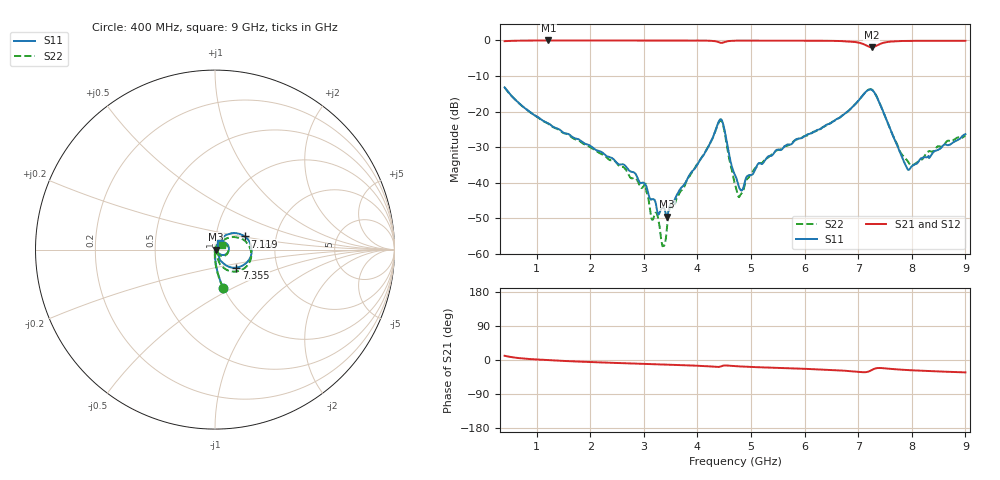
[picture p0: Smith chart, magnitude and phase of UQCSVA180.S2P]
!  Part Number  UQCSVA180  Mounting Orientation: Horizontal
!  Description: Ultra Low ESR Microwave capacitors
!  Application: Coupling, Bypass, Tuning, DC Block
!  Filters, Matching
# GHZ S DB R 50
! Freq  |S11|  S11 Ph  |S21|  S21 Ph  |S12|  S12 Ph  |S22|  S22 Ph
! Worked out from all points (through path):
!   801 points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, 400 MHz to 9 GHz, reference 50 ohm
!   highest |S21| = -0.04 dB at 1.217 GHz (marker M1); lowest = -2.0 dB at 7.248 GHz (marker M2)
!   group delay of S21, straight-line fit = 11.7 ps
!   lowest |S11| = -49.5 dB at 3.432 GHz (marker M3), VSWR 1.01, Z = 50.3 + j0.0271 ohm
!   |S11| at or under -10 dB: start of sweep to end of sweep
!   |S22| runs from -57.8 to -13.2 dB; largest |S21 - S12| = 0.01
!   S11 on the Smith chart (normalised r, x): 400 MHz: 1.00, -0.45; 7.119 GHz: 1.38, +0.21; 7.355 GHz: 1.24, -0.25; 9 GHz: 1.05, +0.08
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0.4  -13.21 -77.5  -0.24 11.2  -0.27 11.2  -13.24 -78.0
1.217  -23.31 -87.4  -0.04 -0.6  -0.08 -0.5  -23.46 -88.2
1.841  -28.44 -89.0  -0.04 -4.5  -0.07 -4.4  -28.75 -91.1
3.012  -40.25 -102.6  -0.04 -10.2  -0.08 -10.1  -40.52 -78.9
3.141  -44.67 -58.1  -0.04 -10.9  -0.07 -10.8  -49.96 -77.9
3.27  -48.93 -34.8  -0.05 -11.4  -0.08 -11.4  -50.38 -41.7
3.356  -47.01 -20.9  -0.05 -11.8  -0.08 -11.8  -57.79 18.0
3.432  -49.50 4.6  -0.05 -12.2  -0.08 -12.2  -52.28 19.3
3.496  -45.90 33.5  -0.04 -12.5  -0.08 -12.5  -46.83 39.8
4.152  -31.22 60.5  -0.09 -16.2  -0.13 -16.1  -31.06 58.8
4.421  -22.23 14.8  -0.66 -17.6  -0.70 -17.5  -22.56 5.7
4.496  -24.55 -30.1  -0.53 -14.6  -0.57 -14.4  -25.02 -41.0
4.7  -37.81 -27.1  -0.10 -16.2  -0.15 -16.0  -40.49 -39.5
4.818  -42.16 16.9  -0.08 -17.1  -0.12 -16.9  -43.03 18.9
5.141  -34.53 60.0  -0.08 -19.1  -0.11 -18.9  -34.73 54.9
6.141  -25.99 64.2  -0.11 -24.1  -0.13 -23.8  -25.87 51.2
7.119  -14.83 23.9  -1.20 -32.3  -1.25 -32.0  -14.84 12.1
7.248  -13.85 -10.2  -1.97 -26.9  -2.02 -26.6  -13.80 -21.7
7.355  -16.19 -40.2  -1.37 -21.3  -1.43 -21.0  -16.11 -51.4
7.57  -23.91 -64.1  -0.42 -23.0  -0.48 -22.6  -23.82 -72.5
7.936  -36.39 -21.3  -0.17 -26.7  -0.21 -26.4  -34.20 -30.8
9  -26.33 54.8  -0.14 -32.7  -0.17 -32.2  -26.67 34.3
